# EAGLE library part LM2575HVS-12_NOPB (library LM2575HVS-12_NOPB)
Texas Instruments, LM2575HVS-12/NOPB Step-Down Switching Regulator 1A, 1.23 57 V, 5-Pin TO-263 Source: Datasheet
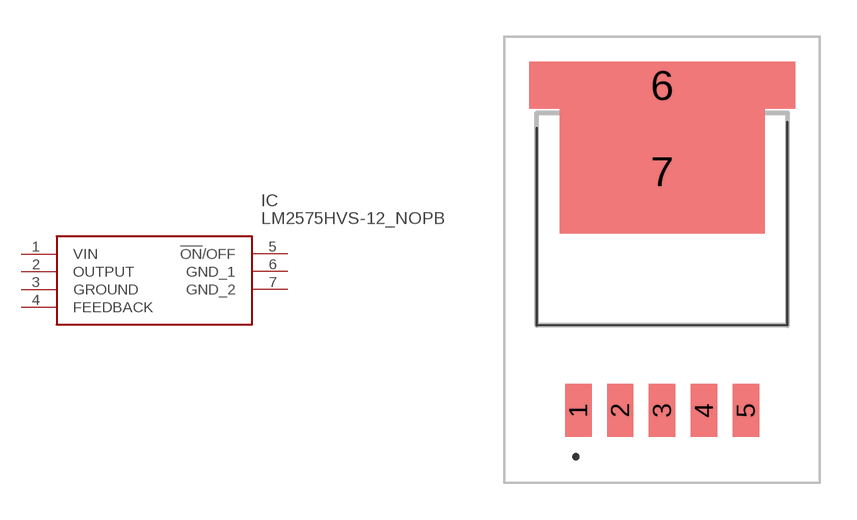
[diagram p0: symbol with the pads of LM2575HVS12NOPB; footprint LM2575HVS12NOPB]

Designator prefix IC

## LM2575HVS-12_NOPB (Description: Texas Instruments, LM2575HVS-12/NOPB Step-Down Switching Regulator 1A, 1.23 57 V, 5-Pin TO-263; Height: 4.65mm; Manufacturer_Name: Texas Instruments; Manufacturer_Part_Number: LM2575HVS-12/NOPB; Mouser_Part_Number: 926-LM2575HVS12NOPB; Mouser_Price-Stock: https://www.mouser.co.uk/ProductDetail/Texas-Instruments/LM2575HVS-12-NOPB?qs=X1J7HmVL2ZEbVPlBGj9cJQ%3D%3D)  [LM2575HVS12NOPB]
1  VIN
2  OUTPUT
3  GROUND
4  FEEDBACK
5  !ON!/OFF
6  GND_1
7  GND_2

## Footprint LM2575HVS12NOPB (pad centres in mm)
LM2575HVS-12/NOPB-3
smd 1.07 x 2.16: 1 -3.4,-7.769; 2 -1.7,-7.769; 3 0,-7.769; 4 1.7,-7.769; 5 3.4,-7.769
smd 10.8 x 1.91: 6 0,5.446
smd 8.33 x 5.08: 7 0,1.95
